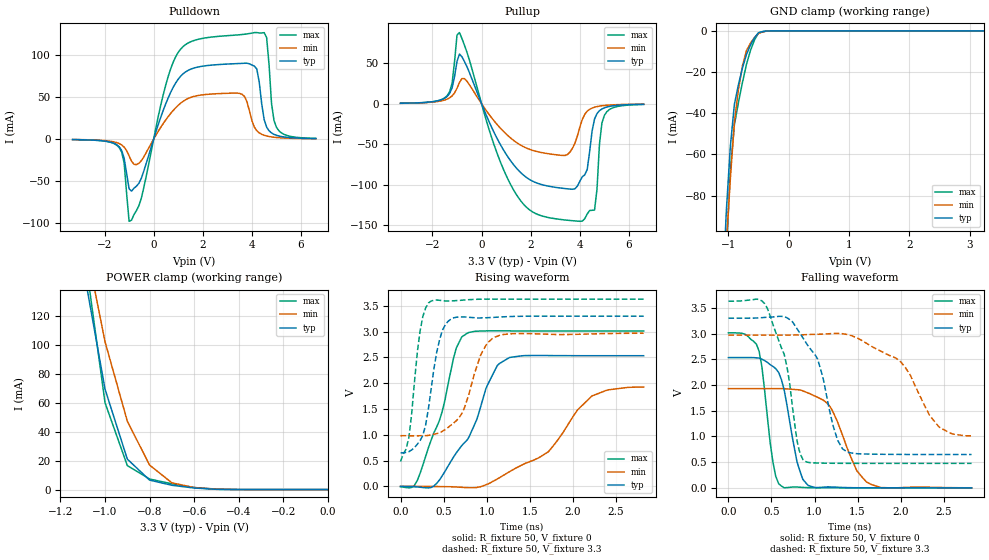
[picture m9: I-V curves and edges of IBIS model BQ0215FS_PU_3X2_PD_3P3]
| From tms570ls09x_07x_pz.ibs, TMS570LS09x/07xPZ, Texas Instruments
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|   Model Cell BQ0215FS_PU_3X2_PD_3P3
|BQ0215FS_PU_3X2_PD_3P3
[Model]   BQ0215FS_PU_3X2_PD_3P3
Model_type   I/O
Polarity   Non-Inverting
Enable   Active-Low
Vinl =  1.25
Vinh =  1.65
Cref =  15.0001pF
Rref =  101.0000M
Vref =  0V
Vmeas =  1.65
C_comp   1.2p   1.2p   1.2p
[Model Spec]
Vinl   1.25   1.12   1.38
Vinh   1.65   1.45   1.75
[Temperature Range]   25   155   -40
[Voltage Range]   3.3   2.97   3.63
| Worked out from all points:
|   slope of the pulldown table from 0 to 0.495 V, typ, clamps not added: 11.8 ohm
|   slope of the pullup table from 0 to 0.495 V, typ, clamps not added: 14.3 ohm
|   GND clamp passes 1 mA (typ) near -0.50 V on its own axis
|   POWER clamp passes 1 mA (typ) near -0.59 V on its own axis
|   rising waveform, R_fixture 50, V_fixture 0: 20-80 % time 435ps typ, 715ps min, 311ps max; typ from 0 V to 2.53 V
|   rising waveform, R_fixture 50, V_fixture 3.3: 20-80 % time 154ps typ, 240ps min, 118ps max; typ from 0.648 V to 3.3 V
|   falling waveform, R_fixture 50, V_fixture 0: 20-80 % time 169ps typ, 283ps min, 125ps max; typ from 2.53 V to 0 V
|   falling waveform, R_fixture 50, V_fixture 3.3: 20-80 % time 299ps typ, 473ps min, 226ps max; typ from 3.3 V to 0.648 V
[POWER_clamp]
|   voltage   I(typ)   I(min)   I(max)
-3.3V     2.375A     2.63A      3.153A
-1.1V     156mA      180.2mA    173.4mA
-1.067V   127.2mA    154.3mA    135.7mA
-1.033V   98.42mA    128.4mA    97.94mA
-1V       69.62mA    102.5mA    60.22mA
-900mV    21.14mA    47.42mA    16.64mA
-800mV    6.593mA    17.01mA    7.345mA
-700mV    3.017mA    4.694mA    4.027mA
-600mV    1.106mA    1.412mA    1.463mA
-500mV    206.7uA    366.5uA    241.6uA
0V        19.75uA    8.576uA    38.26uA
[Pulldown]
|   voltage   I(typ)   I(min)   I(max)
-3.3V     -560.7uA   -504.5uA   -563.6uA
-1.4V     -9.199mA   -5.273mA   -10.11mA
-1.2V     -22.91mA   -9.491mA   -28.67mA
-1V       -59mA      -19.85mA   -97.49mA
-900mV    -61.64mA   -26.24mA   -96.13mA
1V        71.11mA    40.13mA    102.9mA
3.5V      89.74mA    54.24mA    123.8mA
4.2V      83.16mA    9.923mA    126.4mA
4.6V      14.26mA    3.714mA    120.5mA
4.8V      7.317mA    2.617mA    42.02mA
5V        4.531mA    1.939mA    13.99mA
6.6V      631.1uA    487.2uA    853.6uA
[Pullup]
|   voltage   I(typ)   I(min)   I(max)
-3.3V     614.6uA    591.9uA    551.1uA
-1.4V     9.028mA    5.738mA    10.01mA
-900mV    61.32mA    26.24mA    87.8mA
500mV     -34.85mA   -20.79mA   -49.88mA
1.4V      -78.76mA   -47.33mA   -111.2mA
3.4V      -104.6mA   -63.81mA   -143.4mA
4V        -95.71mA   -29.08mA   -145mA
4.3V      -81.25mA   -9.188mA   -136.1mA
4.6V      -18.8mA    -4.29mA    -131.2mA
4.8V      -8.576mA   -2.945mA   -49.93mA
5V        -5.064mA   -2.148mA   -14.33mA
6.6V      -672.1uA   -541.9uA   -866.9uA
[GND_clamp]
|   voltage   I(typ)   I(min)   I(max)
-3.3V     -1.951A    -1.627A    -3.261A
-1.1V     -130.1mA   -138.8mA   -166.7mA
-1.033V   -87.46mA   -103.2mA   -108mA
-966.7mV  -55.98mA   -71.78mA   -67.59mA
-900mV    -35.71mA   -44.42mA   -45.59mA
-833.3mV  -26.16mA   -28.61mA   -34.93mA
-766.7mV  -18.09mA   -17.01mA   -25.16mA
-700mV    -11.51mA   -9.612mA   -16.28mA
-633.3mV  -6.846mA   -5.983mA   -9.513mA
-500mV    -881.4uA   -1.246mA   -1.02mA
-300mV    -7.947uA   -18.83uA   -10.9uA
3.233V    19.75uA    12.58uA    38.26uA
[Ramp]
| variable   typ   min   max
dV/dt_f   1.61425/0.3079601n   1.213519/0.5105585n   1.917722/0.2324539n
dV/dt_r   1.540435/0.442992n   1.17576/0.7393557n   1.826218/0.3139858n
R_load = 50
[Rising Waveform]
R_fixture = 50
V_fixture = 0
V_fixture_min = 0
V_fixture_max = 0
|   time   V(typ)   V(min)   V(max)
0s        -95.2uV    89.34uV    -8.333mV
196ps     -11.57mV   317.9uV    118.4mV
484ps     203.8mV    -5.038mV   1.452V
648ps     649.1mV    -11.6mV    2.684V
776ps     904.2mV    -25.16mV   2.97V
1.124ns   2.343V     142.8mV    3.015V
1.268ns   2.5V       286.9mV    3.015V
1.716ns   2.536V     669.4mV    3.014V
2.224ns   2.533V     1.753V     3.014V
2.824ns   2.533V     1.925V     3.014V
[Rising Waveform]
R_fixture = 50
V_fixture = 3.3
V_fixture_min = 2.97
V_fixture_max = 3.63
|   time   V(typ)   V(min)   V(max)
0s        648.3mV    982.1mV    482.6mV
96ps      671.6mV    981.4mV    937.6mV
260ps     993.3mV    982.5mV    3.298V
356ps     1.892V     999.5mV    3.594V
452ps     2.831V     1.035V     3.608V
548ps     3.194V     1.136V     3.594V
712ps     3.285V     1.411V     3.61V
928ps     3.266V     2.532V     3.629V
1.08ns    3.277V     2.882V     3.631V
2.824ns   3.3V       2.969V     3.63V
[Falling Waveform]
R_fixture = 50
V_fixture = 0
V_fixture_min = 0
V_fixture_max = 0
|   time   V(typ)   V(min)   V(max)
0s        2.533V     1.929V     3.014V
356ps     2.524V     1.93V      2.657V
516ps     2.363V     1.93V      510.4mV
616ps     2.102V     1.931V     33.9mV
796ps     509.9mV    1.909V     15.04mV
928ps     43.57mV    1.843V     2.98mV
1.192ns   17.03mV    1.549V     106.7uV
1.492ns   1.526mV    329.4mV    49.54uV
1.604ns   657.8uV    112.7mV    25.06uV
2.824ns   97.26uV    1.383mV    -8.179uV
[Falling Waveform]
R_fixture = 50
V_fixture = 3.3
V_fixture_min = 2.97
V_fixture_max = 3.63
|   time   V(typ)   V(min)   V(max)
0s        3.3V       2.97V      3.629V
452ps     3.319V     2.97V      3.491V
648ps     3.329V     2.97V      2.596V
796ps     3.096V     2.974V     926.2mV
884ps     2.867V     2.978V     526.5mV
1.036ns   2.503V     2.986V     482.5mV
1.38ns    694.2mV    2.982V     476.2mV
2ns       649.8mV    2.452V     475.4mV
2.46ns    648.2mV    1.165V     475.5mV
2.824ns   647.9mV    1.012V     475.5mV
